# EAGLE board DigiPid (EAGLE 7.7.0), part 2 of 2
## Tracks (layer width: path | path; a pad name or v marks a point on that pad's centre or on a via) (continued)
DAC0 (continued)
  Top 0.127: U12.14 97.67,50.55 97.02,51.2 88.58,51.2 87.82,51.96 U29.52
DAC1
  Top 0.127: U12.13 97.54,51.2 97.28,51.46 91.9,51.46 90.4,52.96 U29.54
DAC2
  Top 0.127: U12.12 92.02,51.85 90.41,53.46 U29.55
DAC3
  Top 0.127: U29.56 90.42,53.96 91.9,52.48 97.54,52.48 97.56,52.5 U12.11
DAC4
  Top 0.127: U12.10 95.13,53.15 94.72,52.74 92.16,52.74 90.44,54.46 U29.57
DAC5
  Top 0.127: U12.9 97.75,53.8 94.98,56.58 85.76,56.58 84.14,54.96 U29.58
DAC6
  Top 0.127: U12.8 97.61,54.45 95.23,56.83 85.25,56.83 83.88,55.46 U29.59
DAC7
  Top 0.127: U12.7 97.73,55.1 95.74,57.09 84.74,57.09 83.61,55.96 U29.60
DAC8
  Top 0.127: U12.6 97.59,55.75 96,57.34 84.22,57.34 83.34,56.46 U29.61
DAC9
  Top 0.127: U29.62 83.07,56.96 83.71,57.6 96.51,57.6 97.71,56.4 U12.5
DAC10
  Top 0.127: U29.64 83.61,57.96 83.71,57.86 96.77,57.86 97.54,57.09 98.05,57.09 98.1,57.1 U12.4
DAC11
  Top 0.127: U29.65 83.88,58.46 84.22,58.11 97.02,58.11 97.44,57.7 U12.3
DAC12
  Top 0.127: U29.66 84.14,58.96 84.74,58.37 98.05,58.37 U12.2
DAC13
  Top 0.127: U12.1 97.36,59 97.01,58.65 86.09,58.65 85.7,59.04 85.7,60.05 85.3,60.45 81.9,60.45 U29.69
DAC_CLK
  Top 0.127: U12.28 104,59.65 104.6,60.25 104.6,61.75 104.5,61.85 101.5,61.85 101.4,61.75 101.4,57.8 101.95,57.25 101.95,55.61 99.33,52.99 99.33,50.53 98.95,50.15 97.31,50.15 96.51,50.94 88.24,50.94 87.54,51.65 83.25,51.65 82.6,51 81.9,51 U29.50
DAC_SLEEP  (via drill 0.2)
  Top 0.127: U12.15 103.65,50.55 v103.05,51.15 | v99.7,54.5 99.7,58.51 94.46,63.74 92.93,63.74 91.65,65.02 91.65,66.91 86.2,72.36 86.2,83.35 83.4,86.15 83.4,95.9 84.65,97.15 86.5,97.15 87.4,98.05 87.4,100.75 87.51,100.86 90.12,100.86 v90.24,100.74 | v92.45,105.25 92.45,121.6 v92.4,121.65 | v93.55,142.7 93.55,145.75 93.25,146.05 U31.95
  Bottom 0.127: v99.7,54.5 v103.05,51.15 | v92.4,121.65 92.4,134.5 89.3,137.6 89.3,138.45 v93.55,142.7 | v92.45,105.25 92.45,102.95 v90.24,100.74
JTAGEN
  Top 0.127: U29.15 69.71,32.98 J7.8
  Top 0.178: J7.8 68.46,31.46 65,28 R81.1 | R81.1
N$1  (via drill 0.2)
  Top 0.127: U4.5 130.69,102.03 131,102.33 131,102.95 R3.2 130.72,103.33 U4.7 128.9,103.35 128.15,103.35 v127.28,104.22 | R7.1 118.05,103.7 117.5,104.25 117.5,106.45 R4.1 118.1,107 118.1,108.37 118.88,109.15 122.05,109.15 124.8,106.4 v125.1,106.4
  Bottom 0.127: v125.1,106.4 v127.28,104.22
N$2
  Top 0.127: U4.9 130.68,104.62 R6.2 130.12,105.92 U4.11 128.9,105.95 124.85,105.95 121.95,108.85 119.09,108.85 118.6,108.36 118.6,104.45 | R8.1 118.05,101.7 118.6,102.25 118.6,104.45 | R5.1 118.6,104.45
N$3  (via drill 0.2)
  Top 0.127: 101.2,85.95 101.2,85.4 101.55,85.05 101.9,85.05 U7.17 | 101.2,85.95 101.55,86.3 101.9,86.3 U7.19 | U5.7 97.5,98 v97,97.5 | v98.15,96.2 100.5,93.85 100.5,88.9 101.2,88.2 101.2,85.95 | R13.1 85,95.8 86.55,94.25 89.1,94.25 90.3,93.05 v94.15,93.05
  Bottom 0.127: v97,97.5 97,97.35 97.72,96.62 | v98.15,96.2 97.72,96.62 | 97.72,96.62 v94.15,93.05
N$4  (via drill 0.2)
  Top 0.127: U6.3 89.3,92.36 90.33,91.33 92.29,91.33 U6.5 92.55,91.1 v93.35,90.3 | U8.7 U8.6 86.65,109.55 86.65,110.05 87.45,110.85 88.8,110.85 90.05,109.6 90.75,109.6 91.15,109.2 v91.15,107.2 | U5.9 98.5,97.75 v99.65,96.6
  Bottom 0.127: v93.35,90.3 v99.65,96.6 99.65,96.65 95.7,100.6 95.7,105.3 93.8,107.2 v91.15,107.2
N$5  (via drill 0.2)
  Top 0.127: R22.1 80.05,99.75 v77.3,97 | v74.7,97.5 74.25,97.05 U9.42
  Bottom 0.127: v77.3,97 76.8,97.5 v74.7,97.5
N$6
  Top 0.127: R21.1 79.7,98 74.88,93.18 73.73,93.18 73.47,93.44 73.47,94.46 73.75,94.74 U9.43
N$7
  Top 0.127: U9.39 75.75,97.49 76.92,98.67 76.92,100.33 77.26,100.67 77.72,100.67 C36.2
N$8  (via drill 0.25)
  Top 0.25: 8.28,8.01 8.28,7.26 9.28,6.26 9.28,5.03 v9.27,5.02 | 8.28,8.01 8.28,8.72 v8.27,8.73 8.28,8.74 8.28,9.51 6.53,11.26 5.91,10.64 5.91,10.63 v5.77,10.49 5.66,10.39 v4.53,9.26 | 8.28,8.01 4.08,8.01 v4.08,7.01
N$9
  Top 0.127: U9.38 U9.37 76.75,97.8 C36.1 78.38,99.05 79,99.67 79,101.95 R20.1
N$10
  Top 0.127: U9.36 79.6,96 C35.2
N$11
  Top 0.127: R18.1 86,98.05 C34.2 83.95,98 R21.2
N$12
  Top 0.127: R19.1 86,99.95 C34.1 83.95,100 R22.2
N$13  (via drill 0.2)
  Top 0.127: U31.72 104.05,143.25 103.1,144.2 103.1,151.6 100.1,154.6 74.5,154.6 v74.3,154.4
  Bottom 0.127: DIS1.RXD 17.33,142 20,144.67 20,150.33 22.67,153 67.8,153 68.65,152.15 72.05,152.15 v74.3,154.4
N$14
  Top 0.127: U8.2 U8.1 83.93,104.47 R16.1B
N$15
  Top 0.127: U29.4 64.21,39.96 L7.1
N$16
  Top 0.127: R84.4B 51.8,48.56 CONF_DONE.TP 52.49,47.87 58.62,47.87 59.04,47.46 U29.138
N$17  (via drill 0.2)
  Top 0.127: R15.1 105.95,87 | 105.95,87 R14.1 C26.1 C25.1 | 92.05,87 C21.1 92.05,87.62 | 92.05,87 C22.1 | C22.1 C23.1 C24.1 | v105.33,87 105.95,87 | v92.67,87 92.05,87 | U6.2 85.42,93.64 R13.2 84.22,93.27 84.22,90.37 84.92,89.67 85,89.67 | 85,89.67 C29.1 84.72,88.67 84.33,88.67 84,88.33 84,86.33 84.33,86 C22.1 | R17.3A 87.6,89.4 87.33,89.67 85,89.67
  Bottom 0.127: v92.67,87 v105.33,87
N$18
  Top 0.127: U19.1 106.05,31 R51.1
N$19
  Top 0.127: C31.1 88.39,109.05 U8.5 87.91,108.57 87.33,108 82.4,108 R16.1A 82.2,107.53 81.4,106.73 R16.2B
N$20
  Top 0.127: U12.18 106.55,52.5 R25.2 R29.1
N$21
  Top 0.178: U11.2 50.66,26.39 C46.1
N$22
  Top 0.127: C48.2 101.95,50.75 103.05,51.85 U12.17
N$23
  Top 0.127: U12.23 106.8,55.75 C52.2
N$24
  Top 0.127: R27.1 C53.2 | R31.1 112.05,55 C53.2 | U12.22 107.46,55.1 107.78,54.78 107.78,53.5 108.29,52.99 109.57,52.99 111.36,54.78 111.83,54.78 C53.2
N$25  (via drill 0.2)
  Top 0.127: R32.1 112.05,53 C53.1 | R28.2 C53.1 | U12.21 104.78,54.45 v104.96,54.27 | v111.1,52.99 111.94,52.99 C53.1
  Bottom 0.127: v104.96,54.27 109.82,54.27 v111.1,52.99
N$26
  Top 0.178: U22.1 90.46,27.51 C80.2 96,28.05 L4.1
N$27
  Top 0.127: R31.2 116.31,54.63 U17.2 121.24,54.63 122.11,53.76 122.11,51.94 R34.1 C62.1
N$28
  Top 0.127: C59.2 R33.2 R32.2 116.31,53.37 U17.3
N$29
  Top 0.178: R61.2 160.55,68 J3.UPR-CTR
N$30
  Top 0.127: C33.1 89.62,106.33 87,106.33 86.64,105.97 U8.3 86.64,103.36 86.67,103.33 86.33,103 R20.2 | R20.2
N$31
  Top 0.127: U31.30 92.75,128.2 C136.2 92.95,128 92.16,128 91.16,127 L8.2
N$32
  Top 0.127: U12.24 105.04,56.4 106.5,57.86 106.91,57.86 C47.1 | C51.2 108.82,54 108.03,54.78 108.03,57.6 107.78,57.86 107.19,57.86 C47.1 | L1.2 105.95,59.1 C47.1
N$33  (via drill 0.2)
  Top 0.127: 87.6,86.6 R17.3B 87.6,87.6 88.33,88.33 88.33,88.73 R17.2A | 87.6,86.6 87.33,86.33 85.72,86.33 C29.2 | 97,85 97,86.33 96.99,86.33 U7.6 95.01,86.33 94.33,87 93.33,87 93,87.33 93,88.67 92.67,89 91,89 v90.67,88.67 90.67,87.33 90,86.67 | 97,85 97,83.67 | 97,83.67 97,82.67 | 97,82.67 101,82.67 | 101,82.67 101,83.33 101.33,83.67 101.87,83.67 U7.15 | U7.13 101.24,82.42 101,82.67 | U7.12 96.76,82.42 97,82.67 | U7.10 96.94,83.72 97,83.67 | U7.8 96.97,85.03 97,85 | 90,86.67 | 90,86.67 89.67,86.33 87.87,86.33 87.6,86.6 | R18.2 87.95,95.39 U6.1 89.09,94.91 v89.33,94.67
  Bottom 0.127: v89.33,94.67 89.33,90 v90.67,88.67
N$34  (via drill 0.2)
  Top 0.127: R2.2 134.53,107.47 | 134.53,107.47 134.32,107.27 D2.A 133.32,105 R6.1 | R10.2 R12.1 103,99 v103.83,99.83 | v106.45,102.45 109.95,102.45 117.25,109.75 122.35,109.75 124.35,107.75 134.25,107.75 134.53,107.47
  Bottom 0.127: v106.45,102.45 v103.83,99.83
N$35
  Top 0.127: R17.2B 88.4,87.73 89.2,88.53 R17.1A 89.33,88.93 89.33,89.33 89.67,89.67 94,89.67 94.33,90 94.33,91.67 93.64,92.36 U6.6
N$36
  Top 0.127: R17.1B 90,88 90,89 90.33,89.33 94.33,89.33 94.67,89.67 94.67,93.33 94.36,93.64 U6.7 92.5,93.65 92,93.65 89.2,96.45 89.2,98.05 87.95,99.3 R19.2
N$37
  Top 0.178: R1.1 156,101 158.67,103.67 162.76,103.67 J1.LWR-CTR
N$38
  Top 0.178: R2.1 149.33,108 150.67,106.67 159.88,106.67 J1.UPR-CTR
N$39
  Top 0.127: R1.2 134.32,101.73 D1.A R3.1 132.95,103.05 132.4,103.6 132.4,106.96 131.91,107.45 124.25,107.45 122.25,109.45 117.35,109.45 109.9,102 R11.1 R9.2
N$40  (via drill 0.2)
  Top 0.127: U31.35 95.25,128.9 92.95,126.6 90.35,126.6 88.7,124.95 v83.4,124.95 | v73.5,131.65 73.5,136.5 68.6,141.4 68.6,148.05 v70.95,150.4 | v72.75,152.2 71.28,153.67 3.33,153.67 1.33,151.67 1.33,70 8.87,62.46 SW4.SW1 12.51,62.46
  Top 0.178: 12.51,62.46 R96.1
  Bottom 0.127: v73.5,131.65 80.2,124.95 v83.4,124.95 | v72.75,152.2 v70.95,150.4
N$41  (via drill 0.2)
  Top 0.127: U19.5 105.4,33.35 v105.22,33.54 | v104.45,34.56 104.39,34.56 R47.2
  Bottom 0.127: v105.22,33.54 105.22,33.79 v104.45,34.56
N$43
  Top 0.127: U5.1 99.65,103.4 R11.2
N$44
  Top 0.127: U5.10 100.65,98.6 R12.2
N$45
  Top 0.127: U7.20 103.03,86.97 R15.2
N$46
  Top 0.127: U7.18 103.72,85.67 R14.2
N$47
  Top 0.127: U7.16 103.67,84.38 C26.2
N$48
  Top 0.127: U7.14 102.97,83.08 C25.2
N$49
  Top 0.127: U7.11 95.03,83.08 C24.2
N$50  (via drill 0.2)
  Top 0.127: U29.32 78.21,41.09 v78.34,40.96
  Bottom 0.127: v78.34,40.96 78.34,38.91 79.1,38.14 82.69,38.14 83.83,37 TP1.TP
N$51  (via drill 0.2)
  Top 0.127: U29.33 78.71,41.35 v79.36,40.7
  Bottom 0.127: v79.36,40.7 80.06,40 TP2.TP
N$52
  Top 0.127: U7.9 94.33,84.38 C23.2
N$53
  Top 0.127: U7.7 94.28,85.67 C22.2
N$54
  Top 0.178: R73.2 154.05,31 | 154.05,31 R74.2 | U28.4 154,31.05 154.05,31
N$55
  Top 0.178: R70.2 R72.2 153,26 151.05,24.05 U27.4
N$56
  Top 0.178: R73.1 163.09,30 J6.LWR-CTR
N$57
  Top 0.178: R70.1 160.55,28 J6.UPR-CTR
N$58  (via drill 0.71)
  Top 0.5: F1.2B F1.2A | F1.2A C1.+VE | F1.2A 27,78 21,84 | 21,84 PWR1.+VIN v21,87.67 | C5.1 20.95,83.95 21,84 | C2.1 33,118.95 | 33,118.95 26.49,118.95 U1.1 | C3.1 26.49,139.95 U2.1 | C4.1 37.41,103.95 U3.3 37,105 | 37,105 37,109.33 33.05,113.28 33.05,118.9 33,118.95 | v21,87.67 | v36,105 37,105
  Bottom 0.5: U1.1 25.21,118.46 23.67,120 23.67,137.13 U2.1 | v36,105 21,90 v21,87.67
N$60  (via drill 0.2)
  Top 0.127: R76.2 141.05,25.8 141.6,26.35 141.6,32.75 133.75,40.6 v117.45,40.6 | v107.5,41.05 86.45,41.05 v84.4,43.1 | v83.05,44.45 82.55,44.95 81.9,44.95 U29.38
  Bottom 0.127: v117.45,40.6 116.1,41.95 108.4,41.95 v107.5,41.05 | v83.05,44.45 v84.4,43.1
N$61  (via drill 0.2)
  Top 0.127: R78.2 141.1,32 133.15,39.95 v117.45,39.95 | v108.6,41.5 92.35,41.5 v87,46.85 | v86.35,47.5 83.6,47.5 82.6,46.5 81.9,46.5 U29.41
  Bottom 0.127: v117.45,39.95 115.9,41.5 v108.6,41.5 | v86.35,47.5 v87,46.85
N$62
  Top 0.178: R69.2 154.05,46.72 150.33,43 149.4,43 U26.4
N$63
  Top 0.178: R65.2 154.05,50 | 154.05,50 R67.2 | U25.4 154,50.05 154.05,50
N$64
  Top 0.178: R69.1 160,47 160.33,46.67 162.76,46.67 J5.LWR-CTR
N$65
  Top 0.178: R65.1 160.55,49 J5.UPR-CTR
N$66  (via drill 0.2)
  Top 0.127: U26.3 135.18,43.05 133.58,41.45 116.76,41.45 116.48,41.73 v116.48,43.52 | v107,44.5 95.7,44.5 92.4,47.8 v87.85,47.8 | v86.95,48.7 82.8,48.7 82.6,48.5 81.9,48.5 U29.45
  Bottom 0.127: v107,44.5 107.95,43.55 116.45,43.55 v116.48,43.52 | v86.95,48.7 v87.85,47.8
N$67  (via drill 0.2)
  Top 0.127: U25.3 140.02,50.05 135.92,45.95 126.08,45.95 123.65,43.52 117.32,43.52 v116.43,44.41 | v108.25,44 107.45,44 107.35,43.9 95.9,43.9 92.5,47.3 v87.45,47.3 | v86.8,47.95 81.9,47.95 U29.44
  Bottom 0.127: v116.43,44.41 116.01,44 v108.25,44 | v86.8,47.95 v87.45,47.3
N$68
  Top 0.127: U7.5 94.97,86.97 C21.2
N$69
  Top 0.127: U15.2 109.33,46.35 109.31,46.34 107.26,46.34 106.75,46.85 106.1,46.85 C57.1
N$70
  Top 0.127: R29.2 108.67,49.73 U15.3 U15.4
N$71
  Top 0.127: U4.20 120.97,102.03 R8.2
N$72
  Top 0.127: U4.18 120.28,103.33 R7.2
N$73
  Top 0.127: U4.16 120.33,104.62 R5.2
N$74
  Top 0.127: U4.14 121.74,105.92 120.67,107 R4.2 | R4.2
N$75
  Top 0.127: 45.08,24.77 45.43,24.77 | U11.4 49.36,25.91 48.64,26.62 45.57,26.62 45.06,26.11 45.06,24.94 U14.1
  Top 0.178: U11.3 U11.4 | 45.08,24.77 U14.1
N$76
  Top 0.127: U21.1 C77.1
N$77
  Top 0.127: U19.7 99.45,32.5 R48.2
N$78
  Top 0.127: R35.CW 113.51,27.54 C61.1
N$79
  Top 0.127: U19.6 100.6,33.55 R47.1
N$80
  Top 0.127: U19.10 98.95,31 R49.2
N$81
  Top 0.127: R38.2 129,51.95 R36.2 | R37.1 149.1,76.95 149.1,73.25 153.6,68.75 153.6,67.25 152.6,66.25 145.95,66.25 131.7,52 R36.2 | R36.2 127.74,53.46 127.74,54.31 R39.1
  Top 0.178: TR1.3 148.2,77.85 R37.1
N$82
  Top 0.178: U18.1 135.22,23.73 C71.1
N$83  (via drill 0.2)
  Top 0.127: R35.W 113.5,25 v116.22,22.27 | v128.77,13.06 128.77,12.28 C66.2
  Bottom 0.127: v116.22,22.27 124.93,22.27 128,19.2 128,13.82 v128.77,13.06
N$84
  Top 0.356: C67.2 146.38,17.95 154.33,10 J4.CONDUCTOR | J4.CONDUCTOR
N$85
  Top 0.178: C69.2 U18.6
N$86
  Top 0.178: R23.1 U13.4 100.95,14.65 R24.2
N$87
  Top 0.178: U18.14 133.95,12.62 133.33,12 C66.1 | C66.1
N$88
  Top 0.127: VCO1.2 124.5,12.46 122.11,14.85 122.11,19.97 118.02,24.06 118.02,24.93 C61.2
  Top 0.178: C64.2 123.95,11.79 VCO1.2
N$89
  Top 0.178: U18.12 132.68,15.68 133,16 136.95,16 C67.1
N$90
  Top 0.178: U10.2 95.67,13.99 96,13.67 96,13.05 C45.1
N$91
  Top 0.127: C73.1 L3.1 106.55,31.5 U19.2 104.46,31.5 104.19,31.23 104.19,28.19 C76.2
N$92
  Top 0.127: U10.3 U10.4 97,14.95 97.1,15.05 U13.3
N$93  (via drill 0.2)
  Top 0.25: R45.2 106.91,36 104.45,33.54 104.45,32.77 104.72,32.5 U19.4
  Top 0.356: R45.2 107.05,36.1 108.4,37.45 124.15,37.45 v125.4,36.2 | v127.25,34.35 127.25,34.25 129.3,32.2 129.3,27.75 C71.2
  Bottom 0.356: v127.25,34.35 v125.4,36.2
N$94
  Top 0.178: VCO1.1 124.95,17.87 C55.1 L2.1
N$95  (via drill 0.2)
  Top 0.127: U31.27 91.25,130.05 90.95,129.75 v85.05,129.75 | v76.15,131.65 76.15,138.15 74.73,139.57 74.73,148.22 v70.35,152.6
  Top 0.178: SW1.B R90.1 13.05,27.61
  Bottom 0.127: v85.05,129.75 84.75,130.05 77.75,130.05 v76.15,131.65 | v70.35,152.6 72.1,152.6 72.9,153.4 72.9,154 3,154 1,152 1,33 SW1.B
N$96
  Top 0.127: U24.12 124.32,33.32 124.1,33.1 123.2,33.1 122.4,33.9 122.15,33.9 C85.2
N$97
  Top 0.356: U24.14 123.6,32.05 122.88,32.77 122.18,32.77 C81.1
N$98  (via drill 0.2)
  Top 0.356: U24.1 132.67,30.78 v133.38,31.49 | v152.06,65.02 153.03,65.02 C89.2
  Bottom 0.356: v133.38,31.49 133.38,46.34 v152.06,65.02
N$99  (via drill 0.2)
  Top 0.127: U19.3 v103.94,32 | v129.02,54.02 129.02,54.93 R39.2 131.04,57.09 134.59,57.09 v142.05,64.55 | TR1.1 144,86 142.05,84.05 v142.05,78.45
  Bottom 0.127: v142.05,78.45 v142.05,64.55 | v103.94,32 103.94,39.42 107.26,42.75 117.76,42.75 v129.02,54.02
N$100
  Top 0.356: C89.1 158.67,65 159.33,65.67 162.76,65.67 J3.LWR-CTR
N$101
  Top 0.178: J2.UPR-CTR TR1.6
N$102
  Top 0.178: R86.1 TP4.TP
N$103
  Top 0.178: VCO1.8 105.49,12.46 C54.1 104.95,15 R26.2
N$104
  Top 0.178: R26.1 R23.2 102.05,16 100.33,16 99.38,16.95 U13.1
N$105
  Top 0.127: U17.6 125.69,53.37 125.83,53.23 | 125.83,53.23 R36.1 125.95,50.9 R34.2 C62.2 | R61.1 142.87,68 132.92,58.05 126.8,58.05 125.85,57.1 125.85,53.25 125.83,53.23
N$106
  Top 0.178: U16.4 47.68,19.62 R30.2 C56.1
N$107  (via drill 0.2)
  Top 0.127: U31.33 94.25,131.45 93.5,132.2 87.2,132.2 v86.65,131.65 | v77.35,131.75 77.35,139.08 76.35,140.08 76.35,149.5 v72.3,153.55
  Top 0.178: SW1.E 10.5,24.5 12,23 14,23 14.95,23.95 R91.1
  Bottom 0.127: 72.2,153.67 3.33,153.67 1.33,151.67 1.33,35.27 9.47,27.14 9.47,24.63 SW1.E | 72.2,153.67 72.33,153.67 | v86.65,131.65 85.65,130.65 78.45,130.65 v77.35,131.75 | v72.3,153.55 72.2,153.65 72.2,153.67
N$108  (via drill 0.2)
  Top 0.127: C77.2 110.08,31.97 110.08,31.23 108.95,30.1 R51.2 108.9,30 107.75,28.85 v104.9,28.85 | v102.25,31.5 U19.9
  Bottom 0.127: v104.9,28.85 v102.25,31.5
N$109
  Top 0.127: L5.2 R59.1
N$110
  Top 0.356: C81.2 L5.1 119.73,31.05 118.78,32 U21.3
N$111
  Top 0.178: R85.1 TP3.TP
N$112  (via drill 0.2)
  Top 0.127: U31.22 84.89,134.25 v84.74,134.4
  Top 0.178: C122.2 TP8.TP
  Bottom 0.127: v84.74,134.4 74.6,134.4 TP8.TP
N$113  (via drill 0.2)
  Top 0.127: U31.23 84.85,133.75 v84.74,133.63
  Top 0.178: C121.2 TP7.TP
  Bottom 0.127: v84.74,133.63 72.37,133.63 TP7.TP
N$114  (via drill 0.2)
  Top 0.127: U31.24 85.12,133.25 v84.74,132.86
  Bottom 0.127: v84.74,132.86 84.48,132.86 83.97,133.38 70.7,133.38 P1.5
N$115  (via drill 0.2)
  Top 0.127: U31.25 85.9,132.75 v85.5,132.35
  Bottom 0.127: v85.5,132.35 84.48,132.35 83.71,133.12 68.42,133.12 P1.4
N$116  (via drill 0.2)
  Top 0.127: U31.21 87.71,134.75 87.55,134.91 v84.22,134.91
  Top 0.178: C124.2 TP9.TP
  Bottom 0.127: v84.22,134.91 77.09,134.91 TP9.TP
N$117  (via drill 0.2, 0.2 pad 0.2)
  Top 0.127: U31.18 95.94,136.25 v96,136.19 | U32.8 137.71,137.75 137.22,138.24 133.38,138.24 v132.61,137.47
  Bottom 0.127: v96,136.19 96.26,135.94 102.4,135.94 105.98,132.35 125.44,132.35 130.56,137.47 v132.61,137.47
N$118  (via drill 0.2, 0.2 pad 0.2)
  Top 0.127: U31.19 95.42,135.75 v95.49,135.68 | U32.7 137.72,138.25 137.47,138.5 132.35,138.5 131.84,137.98 v131.84,136.7
  Bottom 0.127: v95.49,135.68 102.14,135.68 105.73,132.1 125.7,132.1 130.3,136.7 v131.84,136.7
N$119  (via drill 0.2)
  Top 0.127: 131,141.05 131,134 132.33,132.67 137.67,132.67 138,133 138,136.33 138.42,136.75 U32.10 | U31.1 89.55,144.75 v94.6,139.7 | v103.55,145.4 103.8,145.4 105.55,147.15 126.1,147.15 v126.37,146.88 | v130.9,141.58 131,141.48 131,141.05 | 131,141.05
  Bottom 0.127: v94.6,139.7 97.85,139.7 v103.55,145.4 | v126.37,146.88 130.9,142.35 v130.9,141.58
N$120
  Top 0.127: U32.17 141.75,132.08 140,130.33 122.91,130.33 120.06,127.49 118.53,127.49 118.27,127.74 107.52,127.74 107.26,127.49 103.17,127.49 101.25,129.41 U31.47
N$121  (via drill 0.2)
  Top 0.127: U32.18 142.25,131.92 140.33,130 123.09,130 120.32,127.23 118.27,127.23 118.02,127.49 107.78,127.49 107.52,127.23 v102.66,127.23 | U31.48 101.75,129.67 v101.89,129.54
  Bottom 0.127: v102.66,127.23 102.66,128.77 v101.89,129.54
N$122
  Top 0.127: U32.16 141.25,132.25 139.67,130.67 125,130.67 123,132.67 123,140.67 122.35,141.31 106.75,141.31 106.19,140.75 U31.67
N$123
  Top 0.127: U19.8 C74.1 97.28,32 97.02,31.74 97.02,28.42 97.28,28.16 97.79,28.16 L4.2 C76.1
N$124  (via drill 0.2)
  Top 0.127: U32.13 139.75,132.75 138.67,131.67 127.33,131.67 126,133 v126,139.67 | U31.70 106.07,142.25 106.75,141.57 123.65,141.57 124,141.22 v124,139.67
  Bottom 0.127: v124,139.67 v126,139.67
N$125
  Top 0.127: U32.12 138.75,135.75 138.67,135.67 138.67,132.33 138.33,132 131.67,132 127,136.67 R105.2 | R105.2 | R105.2 | U31.71 106.08,142.75 107.01,141.82 126.72,141.82 127,141.54 R105.2
N$126  (via drill 0.2)
  Top 0.127: U32.11 138.58,136.25 138.33,136 138.33,132.67 138,132.33 132,132.33 129,135.33 129,141 127.9,142.1 116.55,142.1 116.4,142.25 116.4,144.95 114.5,146.85 105.65,146.85 103.8,145 103.8,144.95 v103.6,144.75 | U31.12 98.25,139.25 v98.3,139.3
  Bottom 0.127: v98.3,139.3 98.3,139.45 v103.6,144.75
N$127
  Top 0.5: 15V+.TP 24,44 F1.1A F1.1B
N$128
  Top 0.25: C143.1 C142.1 139.75,140.3 U32.6
N$129
  Top 0.127: U32.24 144.92,138.25 147,140.33 R110.2 | R110.2
N$130
  Top 0.127: U32.21 150,136.75 | 150,136.75 155.09,136.75 156.16,135.68 162.12,135.68 P2.1 | R111.2 150,136.75
N$131  (via drill 0.2 pad 0.2)
  Top 0.127: P2.2 157.18,137.82 156,139 156,141.67 154,143.67 R109.2 | R109.2 | U32.20 155.08,136.25 155.9,135.42 159.74,135.42 v160,135.17
  Bottom 0.127: v160,135.17 160,137.37 P2.2
N$132  (via drill 0.2 pad 0.2)
  Top 0.127: P2.3 163,138.33 161,136.33 156.67,136.33 155.2,137.8 | 155.2,137.8 152,141 R108.2 | R108.2 | U32.23 144.87,137.75 v144.9,137.73 | v155.14,137.73 155.2,137.8
  Bottom 0.127: v144.9,137.73 v155.14,137.73
N$133
  Top 0.127: R107.2 | U32.22 145.25,137.25 148,140 R107.2 | P2.6 157.19,146.18 148.74,146.18 148,145.44 R107.2
N$134  (via drill 0.2)
  Top 0.127: C140.1 | C140.1
  Top 0.25: L9.1 C140.1 | C139.1 144,141.05 | 144,141.05 C141.1 142.25,140.3 U32.1 | U32.19 143.92,135.75 v144,135.67 | v144,140.33 144,141.05
  Top 0.253: C140.1 v144,135.67
  Bottom 0.25: v144,135.67 v144,140.33
N$135
  Top 0.127: U32.14 140.25,132.58 139,131.33 127,131.33 125,133.33 R104.2
N$136  (via drill 0.2)
  Top 0.127: U31.55 106.75,134.75 108,136 C127.2 | C127.2 | C127.2 109.76,136 110.08,135.68 110.08,128.77 110.34,128.51 118.02,128.51 118.27,128.77 v120.06,128.77 | v121.6,127.23 151.81,127.23 154.04,125 R98.1
  Bottom 0.127: v120.06,128.77 v121.6,127.23
N$137  (via drill 0.2)
  Top 0.127: U31.54 108.8,134.25 C125.2 109.46,134 109.82,133.63 109.82,128.51 110.08,128.26 118.27,128.26 118.53,128.51 119.3,128.51 v119.55,128.26 | v121.09,126.72 151.81,126.72 155.53,123 R99.1
  Bottom 0.127: v119.55,128.26 v121.09,126.72
N$138
  Top 0.127: U32.3 141.25,149.58 143.47,151.81 168.19,151.81 172.68,147.32 P2.12
N$139
  Top 0.127: U32.2 141.75,149.42 143.88,151.55 157.95,151.55 172.29,137.22 P2.10
N$140
  Top 0.178: R62.2 160.09,63 J3.UPR-COM
N$141  (via drill 0.2)
  Top 0.127: R113.2 156.25,147.2 v158.21,147.2
  Bottom 0.127: v158.21,147.2 164.61,147.2 167.42,144.38 173.85,144.38 P2.11
N$142  (via drill 0.2)
  Top 0.127: U31.51 105.25,132.75 108,130 C135.1 109.05,128.77 109.82,128 v118.78,128 | v122.11,127.74 151.86,127.74 152.6,127 R97.1
  Bottom 0.127: v118.78,128 120.58,126.21 121.86,126.21 122.11,126.46 v122.11,127.74
N$143
  Top 0.127: P2.9 174.25,134.59 172,132.33 168,132.33 167,131.33 158.62,131.33 R112.2
N$144
  Top 0.178: R30.1 48.93,17.32 U16.3 47.28,18.05 46.67,18.67 42.33,18.67 41.68,19.32 U14.3
N$145
  Top 0.178: J8.2 162.6,119.35 D3.5 161.5,118.83 161,118.33 160,118.33 159,119.33 159,122.95 R99.2
N$146  (via drill 0.2)
  Top 0.127: v160.74,123 160.5,123
  Top 0.178: R98.2 159.33,125 160.5,123.84 160.5,123 D3.3
  Bottom 0.127: J8.3 167,122 166,123 v160.74,123
N$147
  Top 0.178: J2.LWR-CTR 164.09,82.42 158.67,77 R37.2 | R37.2
N$148  (via drill 0.2)
  Top 0.127: 109.08,140.25 R93.2 | U31.66 108.8,140.25 R93.2 | R93.2 109.06,140.54 109.57,141.06 112.64,141.06 v112.9,140.8 | R92.2 50MHZ.TP
  Bottom 0.127: v112.9,140.8 112.9,142.9 50MHZ.TP
N$149
  Top 0.178: R87.1 TP5.TP
N$150
  Top 0.178: R88.1 TP6.TP
N$172
  Top 0.178: C88.1 71.64,17.41 U20.10 68.41,17.41 68,17 68,15.05 R46.2
N$173
  Top 0.178: R44.1 R46.1 66,15.05 66,17 65.59,17.41 U20.7 62.36,17.41 R41.1 61.95,15.1 R43.1 R42.2 59.05,13.1 C70.1
N$175
  Top 0.178: R63.2 162.84,13 J4.SHIELD1 164.46,12.54 165,12 165,8 164.46,7.46 J4.SHIELD2
N$193  (via drill 0.2)
  Top 0.127: U31.26 86.85,130.75 85.7,131.9 85.05,131.9 83.75,133.2 v83.75,139.15 | v77,145.9 77,149.56 72.56,154 3,154 1,152 1,38 SW1.A
  Top 0.178: SW1.A 14,32 15,31 15,30.05 R89.1
  Bottom 0.127: v77,145.9 v83.75,139.15
N$194
  Top 0.178: R60.2 161.09,89 J2.LWR-COM
N$195  (via drill 0.2)
  Top 0.127: U31.65 95.2,139.75 89.85,145.1 v84.4,145.1 | v75.6,148 70.55,153.05 69.1,153.05 v68.9,152.85 | 12.51,118.46 SW2.SW1
  Top 0.178: 12.51,118.46 R94.1
  Bottom 0.127: v84.4,145.1 81.5,148 v75.6,148 | v68.9,152.85 68.42,153.33 3.67,153.33 1.67,151.33 1.67,126.67 9.87,118.46 SW2.SW1
N$196  (via drill 0.2)
  Top 0.127: U31.32 93.75,131.45 93.5,131.7 v87.35,131.7 | v77.35,131.1 76.9,131.55 76.9,139.13 76.05,139.98 76.05,148.2 70.92,153.33 3.67,153.33 1.67,151.33 1.67,98 9.54,90.46 SW3.SW1 12.62,91 R95.1
  Bottom 0.127: v87.35,131.7 86,130.35 78.1,130.35 v77.35,131.1
N$197  (via drill 0.2)
  Top 0.127: U31.15 87.83,137.75 87.55,137.47 87.55,137.22 84.99,137.22 v84.74,136.96 | U30.2 61.02,130.98 60.16,131.84 59.39,131.84 58.88,132.35 58.88,134.96 P1.1
  Bottom 0.127: v84.74,136.96 75.78,136.96 71.42,141.31 71.42,142.85 70.91,143.36 60.42,143.36 59.39,142.34 59.39,135.47 P1.1
N$199
  Top 0.127: U12.19 106.2,53.15 C51.1
N$201
  Top 0.178: U28.3 144.95,31.05 144,32 R78.1
N$202  (via drill 0.2)
  Top 0.127: C64.1 68.52,7 v67.07,8.45 | v64.26,11.52 64.26,12.69 R40.2
  Top 0.178: U20.8 64.14,15.19 R43.2 R40.2
  Bottom 0.127: v67.07,8.45 67.07,8.7 v64.26,11.52
N$204  (via drill 0.2)
  Top 0.127: R50.1 77,23.33 | 77,23.33 v77,20 | v77,20 R53.2 | C79.2 87,19 v86,20 | v77,20 | U20.1 67.22,21.22 69.33,23.33 77,23.33
  Bottom 0.127: v86,20 v77,20
N$205  (via drill 0.2)
  Top 0.127: R52.1 v79,22.67 | v79,22.67 R55.2 79.95,18 84.33,18 85,18.67 C82.2 | U20.2 67.25,20.59 69.71,23.04 74.98,23.04 v75.36,22.67 | v79,22.67
  Bottom 0.127: v75.36,22.67 v79,22.67
N$206
  Top 0.178: U23.1 76.05,14.9 C88.2
N$207
  Top 0.178: U27.3 144.95,24.05 144,25 R76.1
N$208
  Top 0.127: U23.5 83.92,11.1 86.33,13.51 86.33,16.38 C79.1
N$209
  Top 0.127: U23.7 84.3,13.63 85,14.33 C82.1 | C82.1
N$210
  Top 0.178: C87.1 70,15 | 70,15 | U20.9 69.86,15.14 70,15 | R44.2 68,13 70,15
N$211
  Top 0.178: TR1.4 160.09,82 J2.UPR-COM
N$212
  Top 0.127: Q1.3 87.33,9.51 86.27,8.45 70.66,8.45 69.38,9.73 63.94,9.73 62.05,11.62
  Top 0.178: R40.1 62.05,11.62
N$213
  Top 0.178: U23.3 75.64,12.37 74,14 74,14.95 C87.2
N$215
  Top 0.127: U31.73 108.3,143.75 R100.1
N$216
  Top 0.178: R71.2 159.09,34 J6.LWR-COM
N$217
  Top 0.178: R68.2 159.09,24 J6.UPR-COM
N$218
  Top 0.178: R66.2 159.09,53 J5.LWR-COM
N$219
  Top 0.178: R64.2 160.09,44 J5.UPR-COM
N$220
  Top 0.127: U31.64 108.3,139.25 108.54,139.01 114.5,139.01 TP12.TP
N$221  (via drill 0.2)
  Top 0.127: U31.56 106.32,135.25 v106.75,135.68
  Bottom 0.127: v106.75,135.68 114.32,135.68 TP11.TP
N$222
  Top 0.127: U31.57 105.8,135.75 107.01,136.96 114.96,136.96 TP10.TP
N$223  (via drill 0.25)
  Top 0.25: v22.48,6.76 20.03,6.76 18.53,5.26 18.53,4.61 v18.58,4.56 | 23.53,4.01 21.83,4.01 v21.78,4.06 v20.98,4.06 20.83,4.06 20.78,4.01 20.03,4.01 20.03,3.01 20.08,2.96 v20.08,2.76 | 23.53,4.01 23.53,3.51 23.48,3.46 v23.48,3.36 | v21.08,5.26 23.28,5.26 23.53,5.01 23.53,4.01 | v18.58,4.56 18.63,4.51 20.33,4.51 v21.08,5.26 | v18.58,4.56 18.53,4.51 18.53,4.01 19.03,3.51 19.28,3.51 19.33,3.46 v19.38,3.46 | 20.96,5.14 v21.08,5.26
N$224  (via drill 0.25)
  Top 0.25: 4.53,2.76 4.53,5.51 4.52,5.53 v4.52,5.75
N$249  (via drill 0.25)
  Top 0.25: v7.54,7.26 5.53,7.26 4.91,6.64 4.89,6.64 v4.76,6.51
N$252  (via drill 0.25)
  Top 0.25: 8.53,2.64 8.53,3.51 8.54,3.52 v8.54,3.76
N$253  (via drill 0.25)
  Top 0.25: 9.78,2.76 9.28,2.76 9.28,3.76 9.53,3.76 9.54,3.77 v9.77,3.77
N$254
  Top 0.25: 9.78,9.26 9.78,7.76 10.03,7.76
N$256  (via drill 0.25)
  Top 0.25: v14.28,9.76 14.28,9.97 14.29,9.98 14.29,9.99 14.29,11.25 14.27,11.27 13.29,11.27 12.92,10.89 12.9,10.89 12.79,10.78 v12.79,10.77
N$257  (via drill 0.25)
  Top 0.25: v6.02,6.51 v6.03,6.51 8.28,6.51 8.28,4.76 8.78,4.26 9.53,4.26 9.76,4.49 v9.78,4.49
N$258  (via drill 0.25)
  Top 0.25: 10.03,5.01 10.03,7.26 9.03,7.26 9.03,9.76 7.16,11.64 7.15,11.64 v7.02,11.77
N$259  (via drill 0.25)
  Top 0.25: v7.53,9.27 7.41,9.39 6.53,10.26 4.78,8.51 3.53,8.51 3.53,3.01 v3.77,3.01
N$260  (via drill 0.25)
  Top 0.25: 3.03,2.89 3.03,8.89 5.91,11.77 v6,11.77
N$261  (via drill 0.25)
  Top 0.25: v12.52,2.76 12.78,2.76 v14.52,2.76 v14.53,2.76 15.9,2.76 16.16,3.01 16.16,3.14 v16.28,3.26 16.28,3.76 16.03,4.01 15.53,4.01
N$262  (via drill 0.25)
  Top 0.25: v20.98,3.26 v22.58,3.26
N$264  (via drill 0.25)
  Top 0.25: v12.28,11.26 12.28,11.52 v12.78,12.02 v12.79,12.01 14.28,12.01 15.13,11.16 15.13,3.51 13.88,3.51 | v12.28,3.77 12.54,3.51 13.88,3.51 | v14.03,8.51 13.88,8.36 13.88,3.51
N$267  (via drill 0.25)
  Top 0.25: 13.41,9.1 14.57,9.1 14.57,4.35 v14.54,4.31 | v13.53,10.51 13.41,10.39 13.41,9.1 | 13.41,9.1 13.41,4.65 v13.03,4.27
N$268  (via drill 0.25)
  Top 0.25: 23.53,8.26 v23.48,8.26 24.08,7.66 24.08,5.96 | v19.48,5.26 19.53,5.26 20.28,6.01 22.43,6.01 v22.48,5.96 22.53,6.01 24.03,6.01 24.08,5.96 | v24.28,3.76 24.28,3.86 24.08,4.06 24.08,5.96
N$270  (via drill 0.25)
  Top 0.25: v22.78,9.26 22.03,8.51 20.78,8.51 20.73,8.46 v20.68,8.46
N$271  (via drill 0.25)
  Top 0.25: v21.68,9.26 20.03,9.26 19.78,9.01 v19.78,8.56 19.78,8.01 20.03,7.76 22.78,7.76 v23.48,7.06
N$273  (via drill 0.25)
  Top 0.25: v24.68,4.36 v24.68,7.16
N$275  (via drill 0.25)
  Top 0.25: v21.08,2.46 21.23,2.46 21.28,2.51 23.43,2.51 v23.48,2.46 23.53,2.51 24.78,2.51 25.28,3.01 25.28,7.51 23.66,9.14 23.66,9.19 v23.58,9.26
N$276  (via drill 0.25)
  Top 0.25: v28.28,5.86 28.28,3.51 28.78,3.01 28.78,2.51
N$277  (via drill 0.25)
  Top 0.25: v28.58,9.26 v31.28,9.26
N$279  (via drill 0.25)
  Top 0.25: v32.58,9.16 32.63,9.16 34.53,7.26 34.53,2.76 34.23,2.46 v33.88,2.46
N$280  (via drill 0.25)
  Top 0.25: v30.38,8.26 32.53,8.26 33.78,7.01 v33.78,3.36
N$281  (via drill 0.25)
  Top 0.25: v32.98,3.16 32.98,3.21 33.03,3.26 33.03,6.76 32.13,7.66 v29.88,7.66
N$283  (via drill 0.25)
  Top 0.25: v27.78,8.96 27.78,8.46 | 27.78,8.46 v27.78,7.76 | 27.78,8.46 27.83,8.51 29.16,8.51 29.28,8.39 29.28,8.01 29.18,7.91 v29.18,7.26
N$284  (via drill 0.25)
  Top 0.25: 28.38,6.76 28.53,6.76 29.03,6.26 29.03,3.76 29.08,3.71 v29.08,3.66 | 28.38,6.76 28.03,6.76 27.53,6.26 27.53,3.26 28.08,2.71 v28.08,2.66 | v28.48,7.96 28.43,7.91 28.43,6.81 28.38,6.76
NCONFIG  (via drill 0.2)
  Top 0.127: U29.129 58.88,51.97 v58.62,51.71 | v52.74,53.25 52.58,53.4 R84.2B
  Bottom 0.127: v58.62,51.71 56.83,53.25 v52.74,53.25
NSTATUS
  Top 0.127: R84.3B 52.87,52.6 53.25,52.22 53.25,50.69 54.02,49.92 57.34,49.92 58.8,48.46 U29.136
PGA-A0  (via drill 0.2)
  Top 0.127: U5.4 97.5,116.8 98.6,117.9 v98.6,124.3 | v97.45,125.45 97.45,129.35 96.75,130.05 U31.38
  Bottom 0.127: v97.45,125.45 v98.6,124.3
PGA-A1  (via drill 0.2)
  Top 0.127: U5.5 97,103.29 93.8,106.49 93.8,120.84 v95.12,122.67 | v101.4,134.55 101.85,134.55 104.05,136.75 U31.59
  Bottom 0.127: v95.12,122.67 95.12,128.27 v101.4,134.55
PHY_50MHZ
  Top 0.127: R92.1 118.17,143 120.32,145.15 138.75,145.15 140.25,143.65 U32.5
RD
  Top 0.127: U31.9 84.08,140.75 82.69,139.35 82.69,123.65 80.9,121.86 63.74,121.86 61.23,119.34 61.23,72.45 64.21,69.47 U29.105
RF_EXT/!INT  (via drill 0.2)
  Top 0.127: Q1.1 89.35,8.7 121.91,8.7 122.89,7.72 122.88,7.71 122.88,5.89 123.39,5.38 125.18,5.38 130.3,10.5 130.3,12.8 130.56,13.06 131.33,13.06 131.33,14.03 131.4,14.1 U18.10 | v106.65,137.25 U31.60 | v109.8,136.45 109.8,136.35 110.4,135.75 110.4,133.25 110.8,132.85 112.85,132.85 v115.68,130.02 | 131.4,14.2 U18.10 | U18.10 131.41,16.21 133.12,17.92 134.52,17.92 140.5,23.9 141.25,23.9 141.9,24.55 141.9,35.15 145.66,38.91 147.66,38.91 154.6,45.85 154.6,61.75 154,62.35 154,68.75 156.93,71.68 165.12,71.68 165.89,72.45 165.89,108.29 151.53,122.65 v123.05,122.65
  Bottom 0.127: v106.65,137.25 109,137.25 v109.8,136.45 | v123.05,122.65 v115.68,130.02
SLO_CLK  (via drill 0.2)
  Top 0.127: U11.6 50.01,21.66 50.33,21.33 55,21.33 v56.33,20 | v96.33,16.33 U10.6 | v95.3,31.62 95.3,32.55 95.6,32.85 96.2,32.85 96.6,33.25 96.6,34.35 99.05,36.8 104.55,36.8 109.05,41.3 109.05,42.75 108.7,43.1 108.7,44.9 U15.6 108.7,44.95 108.7,45.3 109.6,46.2 v111.55,46.2 | v96.35,90.15 96.1,89.9 96.1,89.6 U7.1 | v102.35,91.95 107.35,91.95 108.6,90.7 116.7,90.7 119,93 v119,93.05 | U31.76 102.75,143.9 v103.6,143.05 | v123.3,129.55 121.95,128.2 121.9,128.2 120.6,126.9 120.6,125.44 | v113.4,48.05 113.4,51.65 113.9,52.15 114.5,52.15 114.94,52.59 114.94,55.81 115.97,56.83 115.97,89.34 115.8,89.51 v115.8,89.75 | U4.1 128.93,97.18 124.44,92.7 v123.65,92.7 123.65,90.11 124.42,89.34 134.66,89.34 135.94,90.62 135.94,92.16 136.96,93.18 147.97,93.18 149.76,94.98 164.35,94.98 165.38,96 165.38,108.29 151.3,122.37 123.65,122.37 123.39,122.11 122.88,122.11 120.6,124.39 120.6,125.44 | S-CLK.TP 120.53,125.51 120.6,125.44 | v112.25,140.6 112.56,140.29 113.66,140.29 114.43,141.06 121.34,141.06 122.35,140.05 v122.35,130.5
  Bottom 0.127: v56.33,20 58.67,17.67 95,17.67 95.71,16.96 | 95.71,16.96 v96.33,16.33 | v95.3,31.62 95.3,19.45 96.45,18.3 96.45,17.7 95.75,17 95.71,16.96 | v96.35,90.15 100.55,90.15 v102.35,91.95 | v103.6,143.05 109.8,143.05 v112.25,140.6 | v123.3,129.55 v122.35,130.5 | 123.7,92.7 v123.65,92.7 119.35,92.7 v119,93.05 118.95,93.05 115.8,89.9 v115.8,89.75 | v113.4,48.05 v111.55,46.2
SLO_DAT  (via drill 0.2)
  Top 0.127: U11.7 50.66,22.01 51,21.67 55.33,21.67 v57.33,19.67 | v95.67,18 U10.7 | v93.8,23.75 93.8,25.5 94.1,25.8 95.15,25.8 96.6,27.25 96.6,31.7 96.9,32 96.9,34.25 99.15,36.5 104.65,36.5 109.35,41.2 109.35,44.9 U15.7 109.35,44.95 109.35,45.3 109.65,45.6 112.16,45.6 113.41,46.85 113.97,46.85 115.3,48.18 115.3,55.65 116.25,56.6 116.25,89.9 | v99.48,88.25 96.1,88.25 U7.3 | 116.25,89.9 116.25,89.95 116,90.2 108.13,90.2 v107.71,89.79 | v124.42,92.07 131.6,99.25 131.6,100.75 131.5,100.85 130.6,100.85 130.5,100.75 128.95,100.75 U4.3 128.9,100.75 128.55,100.75 124.05,105.25 v124.05,106.05 | 116.25,89.9 v116.45,89.9 | U31.20 95.25,135.25 97.12,133.38 101.38,133.38 106.75,128 v106.75,127.95 | S-DAT.TP 118.02,119.5 118.02,115.71 124.75,108.98 v125.05,108.98
  Bottom 0.127: v57.33,19.67 59,18 93.8,18 | 93.8,18 v95.67,18 | 93.8,18 v93.8,23.75 | v99.48,88.25 106.18,88.25 v107.71,89.79 | v106.75,127.95 107.31,127.95 112.75,122.51 S-DAT.TP | v125.05,108.98 124.05,107.98 v124.05,106.05 | v124.42,92.07 123.48,92.07 123.14,92.42 118.97,92.42 v116.45,89.9
TCK
  Top 0.127: U29.18 71.21,36.12 72,35.33 75.02,35.33 J7.1
  Top 0.178: J7.1 82.68,34.27 R83.1
TDI  (via drill 0.2)
  Top 0.127: U29.19 71.71,36.62 v72,36.33
  Top 0.178: J7.9 65.27,34.27 63,32 R79.1 | R79.1
  Bottom 0.127: J7.9 67.98,36.33 v72,36.33
TDO  (via drill 0.2)
  Top 0.127: v73.2,35.8 72.2,36.8 U29.20
  Bottom 0.127: v73.2,35.8 73.2,34.6 73.5,34.3 J7.3
TMS
  Top 0.127: U29.16 70.21,35.06 J7.5
  Top 0.178: J7.5 71,33.67 70,32.67 70,30.67 67,27.67 R80.1
TTL1_O/!I!  (via drill 0.2)
  Top 0.127: U31.61 108.25,137.75 v108.3,137.7 | v121.9,130.05 117.25,130.05 113.15,134.14 113.15,135.94 112.79,136.3 v111.7,136.3 | v128.71,123.24 151.45,123.24 166.35,108.34 166.35,65.28 163.07,62 157,62 154.9,59.9 154.9,43.55 147.2,35.85 146.44,35.85 146.18,35.58 146.18,33.79 145.14,33.79 144.2,32.85 142.5,32.85 142.3,32.65 142.3,23.7 R75.2
  Top 0.178: U27.5 149,25 147,23 143,23 R75.2
  Bottom 0.127: v108.3,137.7 110.3,137.7 v111.7,136.3 | v128.71,123.24 v121.9,130.05
TTL2_O/!I!  (via drill 0.2)
  Top 0.127: v96.25,148.4 U31.89 | v119.6,153.75 170.3,153.75 175.6,148.45 175.6,54.1 157.35,35.85 154.35,35.85 150.55,32.05 149.4,32.05 U28.5
  Top 0.178: U28.5 149,32 147,30 142.92,30 R77.2
  Bottom 0.127: v96.25,148.4 101.6,153.75 v119.6,153.75
VCO_MON  (via drill 0.2)
  Top 0.127: R54.1 v81,22 | v81,22 R57.2 | U20.16 70.56,21.22 71.33,22 v73.67,22 | v81,22 | U29.27 75.71,38.29 v76.67,37.33
  Bottom 0.127: v73.67,22 v81,22 81,31.33 76.33,36 76.33,37 v76.67,37.33
WR
  Top 0.127: U31.8 83.92,141.25 82.43,139.76 82.43,123.9 80.64,122.11 63.49,122.11 60.98,119.6 60.98,72.19 63.71,69.46 U29.106

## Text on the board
Top: Design By
tNames: DigiPid / Rev:A, University of Toronto, J.Thywissen Labs
Document: Pentalogix / LAYER STACKUP / ========== / Top 1.7m" Track / pre 7.5m" / 2 1.4m" Ground / pre 4.0m" / 3 1.4m" Power / pre 7.5m" / Bot 1.7m" Track / / Track & Space 5m" (0.127mm) / Drill finished 8m" (0.203mm)
Reference: Connections here | Front view
tDocu: Gain & ADC | Preamp & BW | DAC DC | Move 24MHz net to MCU to edge of board
Target: Alan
